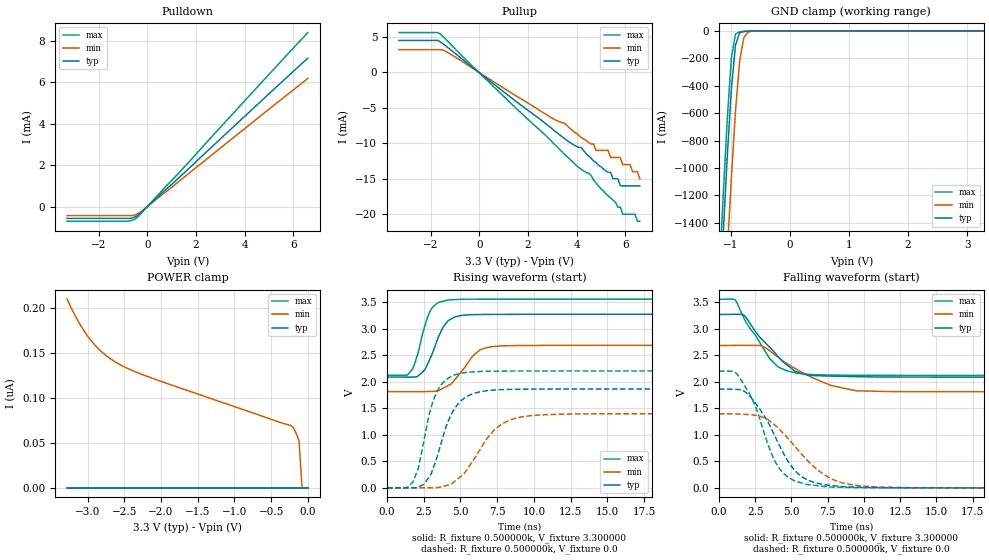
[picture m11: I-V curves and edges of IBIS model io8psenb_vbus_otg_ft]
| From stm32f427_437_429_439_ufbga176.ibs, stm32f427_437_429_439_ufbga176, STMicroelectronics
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|   Model io8psenb_vbus_otg_ft
[Model]  io8psenb_vbus_otg_ft
Model_type 3-state
Polarity   Non-Inverting
Enable   Active-High
Vmeas =  1.650000V
Cref =   50.000000pF
Rref =   100.000000M
Vref =   0.0V
C_comp   3.300900pF   3.198000pF   3.426400pF
[Temperature Range]   25.000000   0.125000k   -40.000000
[Pullup Reference]   3.300000V   2.700000V   3.600000V
[Pulldown Reference]   0.0V   0.0V   0.0V
[POWER Clamp Reference]   3.300000V   2.700000V   3.600000V
[GND Clamp Reference]   0.0V   0.0V   0.0V
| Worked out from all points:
|   slope of the pulldown table from 0 to 0.495 V, typ, clamps not added: 915 ohm
|   slope of the pullup table from 0 to 0.495 V, typ, clamps not added: 372 ohm
|   GND clamp passes 1 mA (typ) near -0.61 V on its own axis
|   rising waveform, R_fixture 0.500000k, V_fixture 3.300000: 20-80 % time 1.09ns typ, 1.48ns min, 877ps max; typ from 2.09 V to 3.27 V
|   rising waveform, R_fixture 0.500000k, V_fixture 0.0: 20-80 % time 1.46ns typ, 2.13ns min, 1.13ns max; typ from 0 V to 1.86 V
|   falling waveform, R_fixture 0.500000k, V_fixture 3.300000: 20-80 % time 2.36ns typ, 3.38ns min, 2.01ns max; typ from 3.27 V to 2.09 V
|   falling waveform, R_fixture 0.500000k, V_fixture 0.0: 20-80 % time 2.3ns typ, 2.98ns min, 1.86ns max; typ from 1.86 V to 0 V
[Pulldown]
|Voltage   I(typ)   I(min)   I(max)
-3.3V     -568.8uA   -435.6uA   -711.6uA
-800mV    -568.8uA   -435.6uA   -711.6uA
-600mV    -538.8uA   -432.7uA   -651.9uA
-400mV    -425uA     -350.3uA   -505.9uA
1.5V      1.61mA     1.403mA    1.882mA
6.6V      7.16mA     6.18mA     8.393mA
[Pullup]
|Voltage   I(typ)   I(min)   I(max)
-3.3V     4.509mA    3.215mA    5.622mA
-1.6V     4.306mA    3.215mA    5.401mA
3.5V      -9.319mA   -7.182mA   -11.52mA
4.7V      -12.5mA    -10.1mA    -15.18mA
4.8V      -12.7mA    -11mA      -15.6mA
5.3V      -14.1mA    -11mA      -17.4mA
5.4V      -14.1mA    -12mA      -17.7mA
5.7V      -15mA      -12mA      -19mA
5.8V      -16mA      -12mA      -19mA
5.9V      -16mA      -13mA      -20mA
6.2V      -16mA      -13mA      -20mA
6.6V      -16mA      -15mA      -21mA
[GND_clamp]
|Voltage   I(typ)   I(min)   I(max)
-3.3V     -9.43A     -9.432A    -9.905A
-1.2V     -2.114A    -2.844A    -1.842A
-1.13V    -1.502A    -2.228A    -1.225A
-1.06V    -927.2mA   -1.634A    -653.4mA
-990mV    -428.8mA   -1.078A    -200.4mA
-920mV    -105.5mA   -587.7mA   -23.3mA
-850mV    -14.69mA   -223.8mA   -6.669mA
-780mV    -4.209mA   -50.78mA   -4.249mA
-710mV    -2.321mA   -9.263mA   -2.64mA
-640mV    -1.305mA   -2.349mA   -1.386mA
3.28V     167.2uA    72.31uA    276.6uA
[POWER_clamp]
|Voltage   I(typ)   I(min)   I(max)
-3.28V    0A         210.1nA    0A
-3.12V    0A         184.2nA    0A
-2.96V    0A         164.6nA    0A
-2.8V     0A         150.7nA    0A
-2.6V     0A         139nA      0A
-2.16V    0A         123.2nA    0A
-240mV    0A         69.7nA     0A
-200mV    0A         67.32nA    0A
-160mV    0A         60.72nA    0A
-120mV    0A         52.23nA    0A
-80mV     0A         0A         0A
0V        0A         0A         0A
[Ramp]
| variable   typ   min   max
dV/dt_r  1.11833/1.45515n   0.83819/2.13142n   1.32215/1.12688n
dV/dt_f  0.71064/2.36020n   0.52386/3.37865n   0.86112/2.00464n
R_load = 0.500000k
[Rising Waveform]
R_fixture= 0.500000k
V_fixture= 3.300000
V_fixture_min= 2.700000
V_fixture_max= 3.600000
|time   V(typ)   V(min)   V(max)
0s        2.088V     1.814V     2.123V
1.376ns   2.087V     1.814V     2.126V
1.752ns   2.088V     1.814V     2.245V
2.503ns   2.205V     1.813V     2.986V
3.128ns   2.563V     1.819V     3.414V
3.754ns   2.996V     1.869V     3.514V
4.254ns   3.166V     1.942V     3.544V
6.381ns   3.268V     2.611V     3.557V
7.758ns   3.271V     2.676V     3.558V
62.31ns   3.272V     2.687V     3.558V
[Rising Waveform]
R_fixture= 0.500000k
V_fixture= 0.0
V_fixture_min= 0.0
V_fixture_max= 0.0
|time   V(typ)   V(min)   V(max)
0s        24.06uV    16.12uV    22.68uV
1.752ns   -592.7uV   -52.48uV   104.4mV
2.503ns   61.6mV     -1.102mV   873.4mV
3.003ns   262.1mV    400.5uV    1.516V
3.504ns   671mV      6.319mV    1.867V
4.379ns   1.388V     69.39mV    2.102V
5.506ns   1.732V     371.4mV    2.18V
7.883ns   1.852V     1.215V     2.2V
10.51ns   1.862V     1.375V     2.203V
62.31ns   1.864V     1.397V     2.204V
[Falling Waveform]
R_fixture= 0.500000k
V_fixture= 3.300000
V_fixture_min= 2.700000
V_fixture_max= 3.600000
|time   V(typ)   V(min)   V(max)
0s        3.272V     2.687V     3.558V
1.126ns   3.275V     2.689V     3.546V
1.752ns   3.254V     2.689V     3.19V
3.003ns   2.791V     2.673V     2.661V
4.004ns   2.504V     2.481V     2.303V
5.255ns   2.201V     2.254V     2.172V
6.256ns   2.12V      2.104V     2.141V
9.384ns   2.099V     1.837V     2.125V
11.89ns   2.091V     1.817V     2.123V
62.31ns   2.088V     1.814V     2.123V
[Falling Waveform]
R_fixture= 0.500000k
V_fixture= 0.0
V_fixture_min= 0.0
V_fixture_max= 0.0
|time   V(typ)   V(min)   V(max)
0s        1.864V     1.397V     2.204V
1.126ns   1.86V      1.395V     2.179V
2.127ns   1.731V     1.381V     1.767V
3.253ns   1.304V     1.304V     925.8mV
4.004ns   896.2mV    1.153V     436.4mV
5.005ns   406.8mV    858.6mV    164.9mV
6.006ns   164.9mV    547.2mV    65.74mV
8.008ns   37.85mV    140.2mV    14mV
10.89ns   5.923mV    17.61mV    405uV
62.31ns   24.06uV    16.12uV    22.68uV
